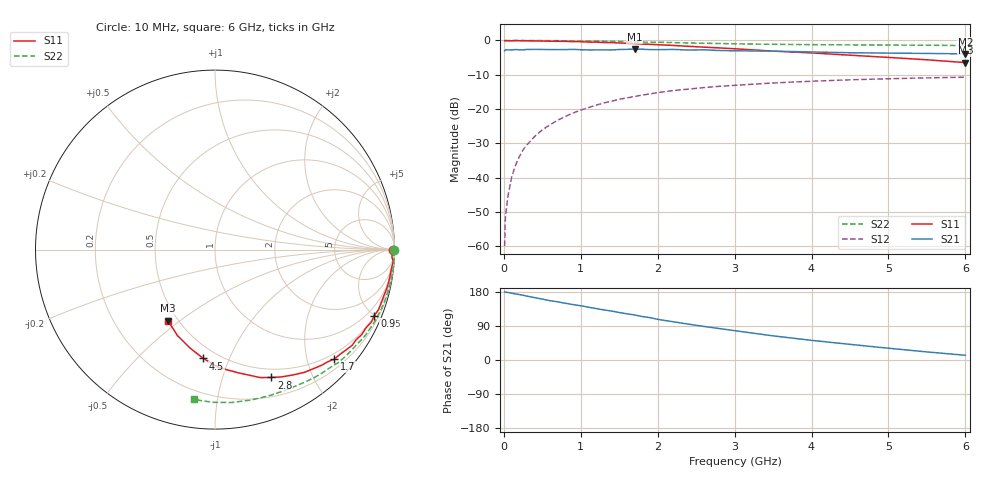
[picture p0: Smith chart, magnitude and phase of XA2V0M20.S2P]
! SIEMENS Discrete & RF Semiconductors
! BFY180
! Si NPN RF Bipolar Junction Transistor in MICRO-X
! VCE = 2 V  IC = 0.2 mA
! Common Emitter S-Parameters:  May  1997
# GHz  S  MA  R  50
!  f  S11  S21  S12  S22
! GHz  MAG  ANG  MAG  ANG  MAG  ANG  MAG  ANG
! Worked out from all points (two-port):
!   36 points, 10 MHz to 6 GHz, reference 50 ohm
!   highest |S21| = -2.53 dB at 1.7 GHz (marker M1); lowest = -3.9 dB at 6 GHz (marker M2)
!   |S21| within 3 dB of the highest: start of sweep to end of sweep
!   lowest |S11| = -6.5 dB at 6 GHz (marker M3), VSWR 2.81, Z = 22.1 - j22.7 ohm
!   |S11| at or under -10 dB: nowhere
!   |S22| runs from -1.5 to 0.0 dB; largest |S21 - S12| = 0.74
!   S11 on the Smith chart (normalised r, x): 10 MHz: open; 900 MHz: 0.52, -4.98; 1.7 GHz: 0.38, -2.52; 2.8 GHz: 0.40, -1.46; 4.5 GHz: 0.42, -0.81; 6 GHz: 0.44, -0.45
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0.01  0.991 -0.2  0.706 180.0  0.001 74.4  0.9999 -0.1
0.02  0.9892 -0.5  0.729 179.0  0.0026 85.6  0.9999 -0.5
0.05  0.9879 -1.0  0.729 178.3  0.0051 85.7  0.999 -1.0
0.1  0.9867 -2.4  0.727 176.3  0.01 89.2  0.9968 -2.1
0.15  0.9948 -3.8  0.737 174.4  0.015 87.3  0.9999 -3.0
0.2  0.9913 -5.2  0.731 172.6  0.0201 86.9  0.9996 -4.1
0.25  0.988 -6.5  0.728 171.0  0.0254 85.0  1 -5.1
0.3  0.9868 -7.6  0.74 168.5  0.0301 83.6  0.9979 -6.0
0.5  0.9814 -12.6  0.739 160.8  0.0496 79.1  0.9953 -10.1
0.7  0.9723 -17.7  0.735 153.5  0.0687 74.8  0.9914 -14.0
0.9  0.9609 -22.5  0.742 146.2  0.0875 70.2  0.9864 -18.1
1.1  0.9469 -27.5  0.727 139.3  0.1049 65.9  0.979 -22.0
1.3  0.933 -32.6  0.729 132.1  0.1227 61.6  0.9718 -26.0
1.7  0.9026 -42.5  0.747 118.8  0.1522 53.4  0.9505 -33.6
2.2  0.8463 -53.9  0.74 101.0  0.1857 43.8  0.9316 -42.6
2.6  0.7989 -62.7  0.73 88.6  0.2055 37.0  0.9106 -49.0
2.8  0.7782 -66.2  0.714 83.0  0.2145 33.7  0.9028 -52.1
3.5  0.6991 -79.2  0.699 63.7  0.2399 23.6  0.8784 -62.3
4  0.658 -88.1  0.679 51.9  0.2543 16.9  0.8686 -69.4
4.5  0.6098 -96.1  0.662 41.3  0.2668 10.8  0.8618 -76.5
5.5  0.5227 -113.6  0.647 21.3  0.2848 -1.1  0.851 -90.9
6  0.4751 -123.4  0.637 12.5  0.2913 -7.1  0.8432 -98.1
